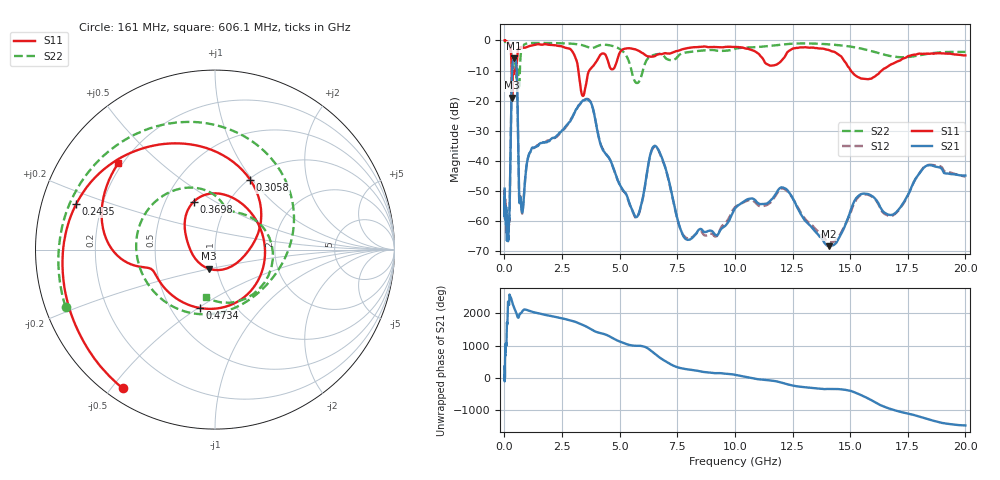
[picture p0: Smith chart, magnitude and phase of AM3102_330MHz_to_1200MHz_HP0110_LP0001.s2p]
! Date/Time: Tue, Sep 11, 2018 5:14 PM
! Network Analyzer: Agilent Technologies E8362B Rev: A.07.50.63
! Sweep from 0.010 to 20.000 GHz, 1601 Points, Sweep Type: LOG
! Power Supply: 4.949 V, 0.001 A
# Hz S DB R 50
!freq MagS11 AngS11 MagS21 AngS21 MagS12 AngS12 MagS22 AngS22
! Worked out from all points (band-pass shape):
!   1601 points, 10 MHz to 20 GHz, reference 50 ohm
!   highest |S21| = -5.99 dB at 424.4 MHz (marker M1); lowest = -68.3 dB at 14.07 GHz (marker M2)
!   |S21| within 3 dB of the highest: 340.9 MHz to 527.3 MHz (186.3 MHz wide, 42.9 % of centre)
!   lowest |S11| = -19.0 dB at 337.9 MHz (marker M3), VSWR 1.25, Z = 45.8 - j9.94 ohm
!   |S11| at or under -10 dB: 315 MHz to 453.8 MHz (138.8 MHz wide, 36.1 % of centre); 3.207 GHz to 3.681 GHz (473.6 MHz wide, 13.8 % of centre); 15.03 GHz to 16.37 GHz (1.341 GHz wide, 8.54 % of centre)
!   |S22| runs from -16.2 to -0.2 dB; largest |S21 - S12| = 0.0067
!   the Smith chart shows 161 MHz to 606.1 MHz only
!   S11 on the Smith chart (normalised r, x): 161 MHz: 0.05, -0.54; 243.5 MHz: 0.11, +0.16; 305.8 MHz: 1.02, +0.98; 369.8 MHz: 0.69, +0.40; 473.4 MHz: 0.69, -0.51; 606.1 MHz: 0.18, +0.37
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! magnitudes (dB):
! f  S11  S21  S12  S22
! 10 MHz  0.0  -49.2  -49.7  -0.2
! 35.55 MHz  0.0  -57.5  -58.7  -0.4
! 126.4 MHz  -0.4  -60.1  -62.4  -0.8
! 161 MHz  -0.6  -65.9  -63.7  -1.0
! 243.5 MHz  -1.8  -48.4  -48.5  -1.9
! 305.8 MHz  -7.2  -18.6  -18.7  -4.9
! 337.9 MHz  -19.0  -9.4  -9.5  -8.7
! 369.8 MHz  -10.7  -6.9  -6.9  -8.9
! 424.4 MHz  -11.1  -6.0  -6.0  -7.2
! 447.2 MHz  -10.2  -6.1  -6.1  -7.1
! 473.4 MHz  -9.5  -6.3  -6.4  -7.8
! 543.4 MHz  -7.0  -11.8  -11.9  -12.3
! 606.1 MHz  -2.8  -38.1  -38.2  -11.4
! 772.3 MHz  -2.4  -57.0  -57.5  -2.3
! 1.59 GHz  -1.4  -34.0  -34.1  -0.8
! 3.634 GHz  -10.8  -19.7  -19.5  -2.3
! 5.652 GHz  -2.9  -58.1  -58.4  -13.5
! 6.58 GHz  -4.9  -35.2  -35.4  -4.6
! 7.92 GHz  -2.6  -66.1  -65.6  -3.9
! 12.03 GHz  -6.6  -48.7  -49.1  -1.4
! 14.07 GHz  -3.2  -68.3  -66.8  -1.3
! 20 GHz  -4.9  -44.8  -45.2  -3.8
